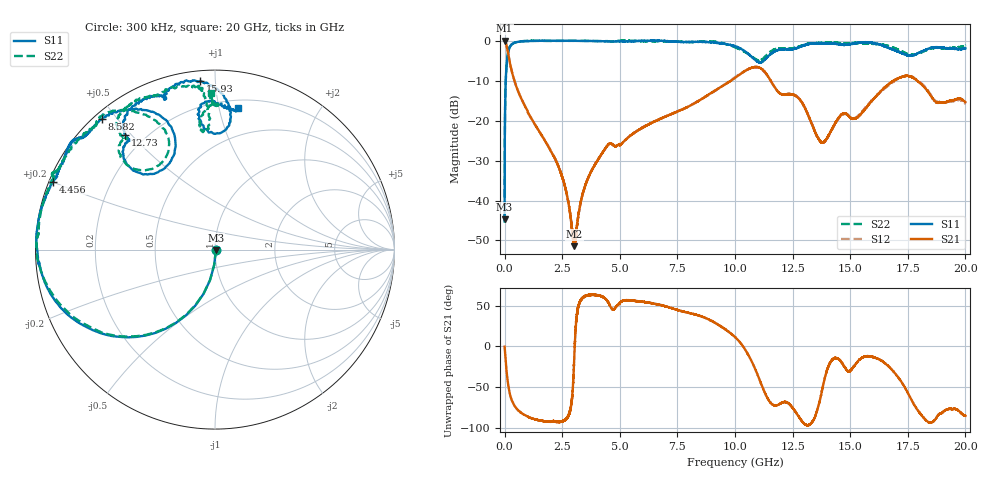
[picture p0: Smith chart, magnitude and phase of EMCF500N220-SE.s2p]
!EMCF500N220
!Johanson Technology Inc.
!www.johansontechnology.com
!Test Board Conditions:
!Substrate Type  RO4350B
!Substrate Thickness  6.6 mil
!Substrate Dk  3.66
!TL Type: GCPW
!TL Trace Width  13 mil
!TL Gap  7.5 mil
!PART MODE SINGLE ENDED (AKA BYPASS)
!DUT TOPOLOGY	SERIES-SHUNT
# MHz S  dB  R 50
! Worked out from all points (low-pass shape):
!   20001 points, 300 kHz to 20 GHz, reference 50 ohm
!   highest |S21| = -0.01 dB at 300 kHz (marker M1); lowest = -51.4 dB at 3.031 GHz (marker M2)
!   |S21| within 3 dB of the highest: start of sweep to 145.8 MHz
!   lowest |S11| = -44.7 dB at 300 kHz (marker M3), VSWR 1.01, Z = 50.6 - j0.187 ohm
!   |S11| at or under -10 dB: start of sweep to 49.93 MHz
!   |S22| runs from -45.5 to 0.0 dB; largest |S21 - S12| = 0.011
!   S11 on the Smith chart (normalised r, x): 300 kHz: 1.01, -0.00; 4.456 GHz: 0.01, +0.20; 8.582 GHz: 0.02, +0.46; 12.73 GHz: 0.13, +0.48; 15.93 GHz: 0.05, +0.91; 20 GHz: 0.26, +1.14
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0.3  -44.72 -18.5  -0.01 -0.3  -0.01 -0.3  -45.53 -10.9
111.298  -4.51 -127.4  -2.00 -37.3  -1.99 -37.3  -4.58 -127.5
268.296  -1.19 -153.0  -6.62 -62.3  -6.60 -62.5  -1.25 -153.7
1100.284  -0.12 -176.3  -18.89 -87.4  -18.93 -87.2  -0.06 178.9
2396.264  -0.04 169.7  -32.38 -92.5  -32.33 -92.6  -0.08 173.0
3031.255  -0.07 165.4  -51.42 -9.3  -51.07 -9.1  -0.07 167.6
3334.25  -0.07 164.2  -39.60 58.1  -39.61 58.2  -0.06 164.4
4456.233  -0.21 157.2  -26.28 55.9  -26.32 55.8  -0.12 156.5
6667.2  -0.02 142.7  -19.83 51.6  -19.76 51.3  -0.16 147.6
8582.171  -0.33 131.0  -14.51 36.3  -14.53 36.0  -0.24 132.6
10000.15  -1.43 115.0  -9.35 11.6  -9.17 11.6  -1.67 116.4
10735.14  -4.12 110.5  -6.79 -18.9  -6.84 -19.8  -4.02 114.1
11234.13  -5.10 130.8  -7.46 -52.7  -7.57 -52.8  -4.47 132.5
12732.11  -1.80 128.1  -14.28 -84.4  -14.21 -84.5  -1.62 129.4
13334.1  -0.77 120.6  -20.86 -93.2  -20.80 -93.6  -0.70 124.9
13836.09  -0.71 114.4  -25.47 -46.5  -25.49 -46.6  -0.60 121.3
14621.08  -1.06 108.5  -18.51 -19.6  -18.67 -18.5  -0.62 112.7
15925.06  -0.51 95.1  -15.15 -12.7  -15.01 -13.7  -0.73 96.6
16667.05  -1.85 84.8  -10.90 -24.4  -11.23 -24.7  -1.37 93.8
17692.03  -3.66 91.7  -9.16 -67.2  -9.01 -66.3  -3.55 95.6
18749.02  -1.66 91.5  -15.48 -87.2  -15.31 -88.3  -1.79 89.9
20000  -1.93 80.8  -15.43 -85.1  -15.75 -83.9  -1.19 91.2
